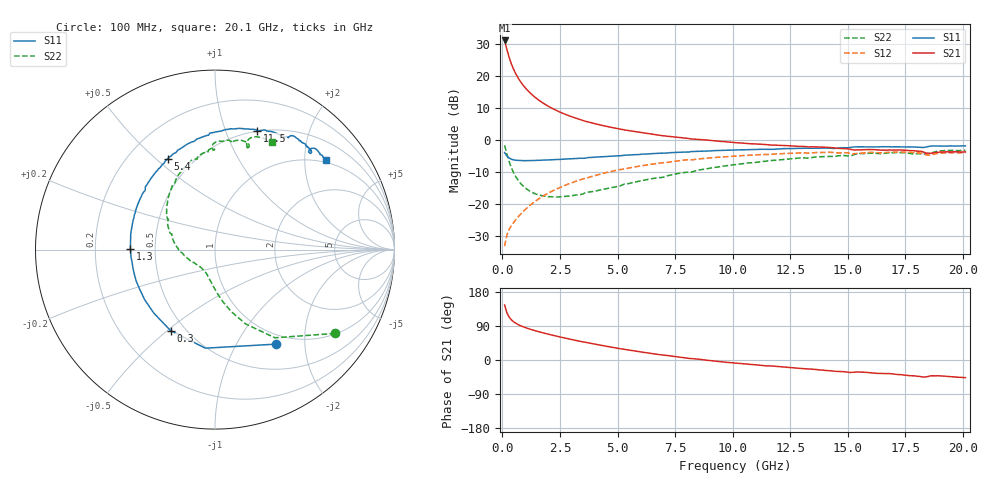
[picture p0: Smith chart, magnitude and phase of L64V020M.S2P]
!  Infineon Technologies AG
! BFR380L3 , PF131585-7, No.6, Th 09.10.01, soldered on pcb-board, measured with PP GSG850
!  Vce=4.0 V,  Ic=20.0 mA
! Common Emitter S-Parameters:  15. November 2001
#  GHz  S  MA  R  50
! f  S11  S21  S12  S22
! GHz  Mag  Ang  Mag  Ang  Mag  Ang  Mag  Ang
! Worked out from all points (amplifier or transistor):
!   201 points, 100 MHz to 20.1 GHz, reference 50 ohm
!   highest |S21| = 31.0 dB at 100 MHz (marker M1)
!   |S21| within 3 dB of that: start of sweep to 206.3 MHz
!   unconditionally stable (mu >= 1): 1.451 GHz to 4.398 GHz
!   at 3.4 GHz: K = 1.02, MAG = 8.5 dB, |S12| = -12.5 dB
!   at 10.1 GHz: K = 0.95, MSG = 2.1 dB, |S12| = -5.2 dB
!   at 20.1 GHz: K = 0.98, MSG = 0.1 dB, |S12| = -4.1 dB
!   S11 on the Smith chart (normalised r, x): 100 MHz: 0.85, -1.47; 300 MHz: 0.42, -0.51; 1.3 GHz: 0.36, +0.00; 5.4 GHz: 0.36, +0.55; 11.5 GHz: 0.50, +1.30; 20.1 GHz: 0.93, +2.54
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0.1  0.6256 -57.4  35.32 145.2  0.02162 63.4  0.8163 -34.9
0.2  0.5519 -95.6  25.47 124.5  0.03253 55.9  0.5939 -55.8
0.3  0.5145 -118.8  19.06 113.0  0.04 54.3  0.4485 -67.6
0.4  0.4915 -133.8  15 105.6  0.04549 54.4  0.3579 -75.3
0.5  0.4813 -144.4  12.3 100.4  0.05108 56.2  0.2987 -80.8
0.6  0.4742 -152.2  10.39 96.4  0.05692 57.6  0.2576 -85.3
0.7  0.4727 -158.5  9.006 93.1  0.06264 58.9  0.2275 -89.2
0.8  0.4698 -163.6  7.929 90.2  0.06873 60.1  0.2054 -92.5
0.9  0.4682 -167.7  7.082 87.8  0.07503 61.0  0.1881 -95.5
1.1  0.4698 -174.8  5.85 83.4  0.08755 62.3  0.1648 -101.3
1.3  0.4715 179.3  4.984 79.5  0.1003 63.0  0.1493 -106.3
1.7  0.4769 169.9  3.855 72.7  0.1265 63.2  0.1332 -115.8
2.1  0.4826 162.1  3.16 66.6  0.1527 62.3  0.1279 -124.4
2.7  0.4957 151.8  2.507 58.2  0.1915 59.9  0.1294 -137.0
3.5  0.5101 140.0  1.986 47.8  0.243 55.6  0.1411 -149.8
5.4  0.5714 117.5  1.396 27.2  0.3528 43.8  0.2037 179.9
6.8  0.6102 103.5  1.172 14.3  0.4281 34.1  0.2543 161.1
10.1  0.6879 78.9  0.8951 -8.0  0.5523 12.6  0.4064 128.3
11.5  0.703 70.3  0.8293 -15.5  0.5838 3.7  0.4645 115.9
13.5  0.7328 61.2  0.7711 -24.4  0.6224 -8.2  0.5263 100.4
16.8  0.7721 48.7  0.6867 -35.8  0.631 -24.3  0.6196 78.9
20.1  0.7958 38.8  0.6424 -46.6  0.6249 -38.2  0.6792 62.4
